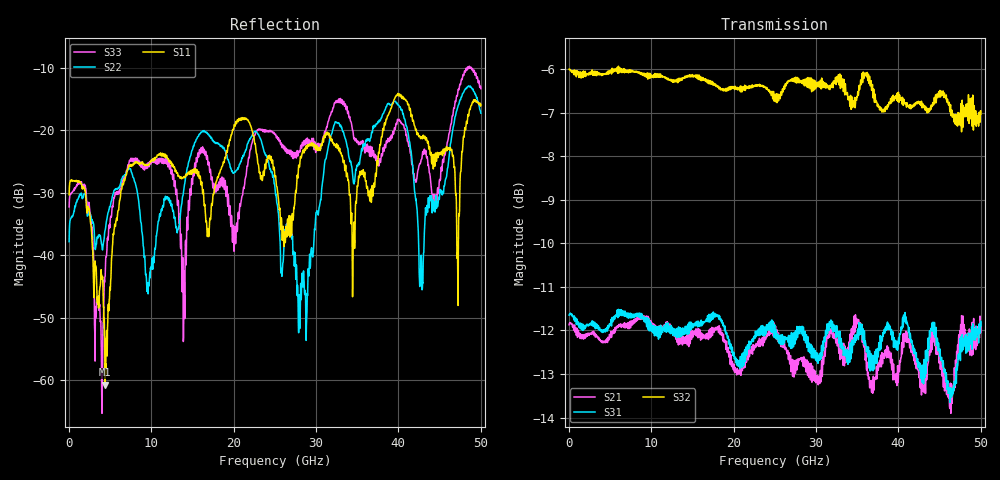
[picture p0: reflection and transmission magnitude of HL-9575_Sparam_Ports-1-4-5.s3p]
# GHZ S RI R 50.0
!; PortSelection: Port_123
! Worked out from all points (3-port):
!   1429 points, 35 MHz to 50.02 GHz, reference 50 ohm
!   strongest paths, dB at 35 MHz, 12.53 GHz, 25.02 GHz, 37.52 GHz, 50.02 GHz:
!     S32: -6.0, -6.3, -6.6, -6.8, -7.0
!     S31: -11.7, -12.0, -12.0, -12.4, -11.9
!     S21: -11.9, -12.1, -12.1, -12.9, -11.9
!   lowest |S11| = -60.7 dB at 4.41 GHz (marker M1), VSWR 1.00, Z = 50.1 + j0.0225 ohm
!   |S11| at or under -10 dB: start of sweep to end of sweep
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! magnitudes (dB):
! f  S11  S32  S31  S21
! 35 MHz  -30.3  -6.0  -11.7  -11.9
! 4.41 GHz  -60.7  -6.1  -12.0  -12.3
! 7.42 GHz  -25.6  -6.1  -11.7  -11.8
! 13.96 GHz  -27.6  -6.2  -12.0  -12.2
! 25.02 GHz  -27.5  -6.6  -12.0  -12.1
! 28.77 GHz  -22.6  -6.4  -12.2  -12.8
! 34.51 GHz  -39.2  -6.8  -12.3  -11.9
! 39.66 GHz  -14.6  -6.7  -12.2  -13.1
! 42.77 GHz  -21.0  -6.8  -12.9  -13.3
! 50.02 GHz  -15.9  -7.0  -11.9  -11.9
